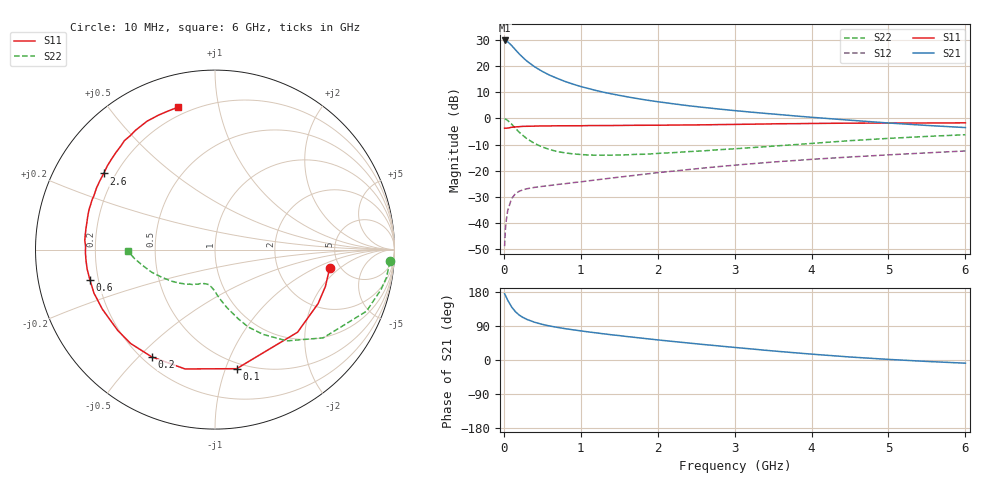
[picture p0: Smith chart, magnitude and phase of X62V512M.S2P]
! SIEMENS Small Signal Semiconductors
! BFP193W
! Si NPN RF Bipolar Junction Transistor in SOT343
! VCE = 2.5 V  IC = 12 mA
! Common Emitter S-Parameters:  April 1994
# GHz  S  MA  R  50
!  f  S11  S21  S12  S22
! GHz  MAG  ANG  MAG  ANG  MAG  ANG  MAG  ANG
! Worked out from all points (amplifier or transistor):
!   40 points, 10 MHz to 6 GHz, reference 50 ohm
!   highest |S21| = 29.8 dB at 10 MHz (marker M1)
!   |S21| within 3 dB of that: start of sweep to 133.7 MHz
!   unconditionally stable (mu >= 1): 1.192 GHz to 4.119 GHz
!   at 200 MHz: K = 0.25, MSG = 26.3 dB, |S12| = -27.9 dB
!   at 1.5 GHz: K = 1.09, MAG = 13.8 dB, |S12| = -22.5 dB
!   at 6 GHz: K = 0.93, MSG = 4.5 dB, |S12| = -12.5 dB
!   S11 on the Smith chart (normalised r, x): 10 MHz: 4.11, -1.48; 100 MHz: 0.45, -1.09; 200 MHz: 0.24, -0.55; 600 MHz: 0.17, -0.12; 2.6 GHz: 0.16, +0.30; 6 GHz: 0.16, +0.76
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0.01  0.6472 -9.3  30.84 174.6  0.0036 88.3  0.9771 -3.8
0.02  0.6485 -18.5  30.75 170.9  0.0074 80.5  0.968 -9.3
0.03  0.6485 -27.6  30.37 166.5  0.0108 78.2  0.951 -13.6
0.05  0.6508 -45.0  29.09 157.9  0.0172 70.5  0.9115 -22.1
0.1  0.6744 -79.7  24.79 140.4  0.0291 56.4  0.7781 -39.2
0.15  0.6856 -104.1  20.52 127.5  0.0362 46.8  0.6471 -51.8
0.2  0.6938 -120.5  17.04 118.6  0.0404 40.8  0.5435 -60.4
0.25  0.7033 -131.9  14.47 112.1  0.0431 37.1  0.4688 -66.8
0.3  0.7047 -140.3  12.41 107.1  0.0451 34.9  0.4071 -71.4
0.4  0.7101 -152.2  9.679 99.6  0.0479 33.2  0.3308 -78.3
0.5  0.7166 -160.3  7.896 94.0  0.0501 33.1  0.2833 -83.4
0.6  0.717 -166.3  6.643 89.6  0.0521 33.5  0.2522 -87.4
0.8  0.7212 -175.1  5.046 82.6  0.0564 36.0  0.2184 -93.0
1.1  0.7272 175.9  3.718 74.1  0.0639 40.1  0.1989 -99.9
1.3  0.7284 170.7  3.151 69.0  0.0694 42.5  0.1976 -103.7
1.6  0.7344 164.0  2.588 61.9  0.0782 45.0  0.2007 -108.9
2.2  0.744 152.6  1.9 48.9  0.0979 47.7  0.2208 -119.4
2.6  0.7513 145.6  1.616 40.8  0.1123 47.9  0.2393 -126.6
3.2  0.7729 135.6  1.32 29.5  0.1346 46.7  0.2744 -137.2
4.5  0.8094 117.9  0.921 7.9  0.1825 41.0  0.3745 -160.3
5.5  0.8149 108.8  0.732 -3.8  0.2187 35.6  0.4513 -173.7
6  0.8201 104.4  0.666 -8.4  0.2382 33.1  0.4866 -179.1
